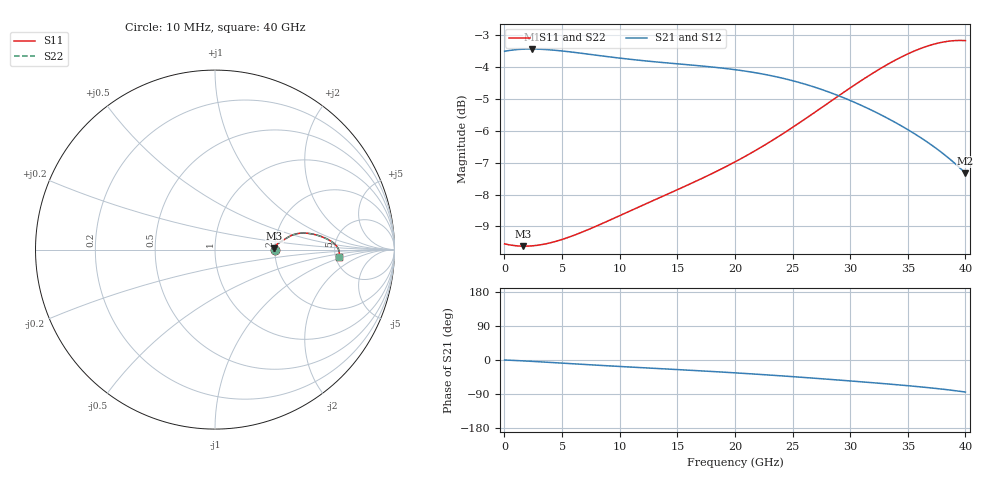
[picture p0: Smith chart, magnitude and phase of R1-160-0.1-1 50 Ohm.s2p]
!version-1
!date-09.2020
# MHz S RI R 50
!Freq ReS11 ImS11 ReS21 ImS21 ReS12 ImS12 ReS22 ImS22
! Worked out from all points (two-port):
!   101 points, 10 MHz to 40 GHz, reference 50 ohm
!   highest |S21| = -3.45 dB at 2.41 GHz (marker M1); lowest = -7.3 dB at 40 GHz (marker M2)
!   |S21| within 3 dB of the highest: start of sweep to 37.05 GHz
!   lowest |S11| = -9.6 dB at 1.61 GHz (marker M3), VSWR 1.99, Z = 99.3 + j1.77 ohm
!   |S11| at or under -10 dB: nowhere
!   |S22| runs from -9.6 to -3.2 dB; largest |S21 - S12| = 0
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10  0.3333 5.13e-05  0.6667 -0.000147  0.6667 -0.000147  0.3333 5.13e-05
1610  0.3304 0.00792  0.6712 -0.0272  0.6712 -0.0272  0.3304 0.00792
2410  0.3307 0.0117  0.6707 -0.0427  0.6707 -0.0427  0.3307 0.0117
4410  0.3355 0.0206  0.6638 -0.0835  0.6638 -0.0835  0.3355 0.0206
6810  0.3468 0.0307  0.6481 -0.1319  0.6481 -0.1319  0.3468 0.0307
10010  0.3664 0.0437  0.6218 -0.1909  0.6218 -0.1909  0.3664 0.0437
13610  0.3903 0.0588  0.5896 -0.2502  0.5896 -0.2502  0.3903 0.0588
17210  0.416 0.0738  0.553 -0.306  0.553 -0.306  0.416 0.0738
20010  0.4398 0.084  0.5177 -0.3482  0.5177 -0.3482  0.4398 0.084
21610  0.456 0.0884  0.4936 -0.3715  0.4936 -0.3715  0.456 0.0884
23210  0.4746 0.0912  0.4663 -0.3936  0.4663 -0.3936  0.4746 0.0912
24810  0.4958 0.092  0.4358 -0.4138  0.4358 -0.4138  0.4958 0.092
26810  0.5257 0.0896  0.3934 -0.4353  0.3934 -0.4353  0.5257 0.0896
28810  0.5587 0.0831  0.3471 -0.4518  0.3471 -0.4518  0.5587 0.0831
30410  0.5861 0.0749  0.3082 -0.4609  0.3082 -0.4609  0.5861 0.0749
32010  0.6135 0.0641  0.2679 -0.4661  0.2679 -0.4661  0.6135 0.0641
33610  0.6393 0.0509  0.2267 -0.4675  0.2267 -0.4675  0.6393 0.0509
35610  0.6671 0.0307  0.1732 -0.4638  0.1732 -0.4638  0.6671 0.0307
37210  0.6835 0.0106  0.1279 -0.456  0.1279 -0.456  0.6835 0.0106
38010  0.6889 -0.00126  0.1041 -0.4502  0.1041 -0.4502  0.6889 -0.00126
38810  0.692 -0.0147  0.0793 -0.4427  0.0793 -0.4427  0.692 -0.0147
40000  0.6916 -0.0387  0.0402 -0.4278  0.0402 -0.4278  0.6916 -0.0387
